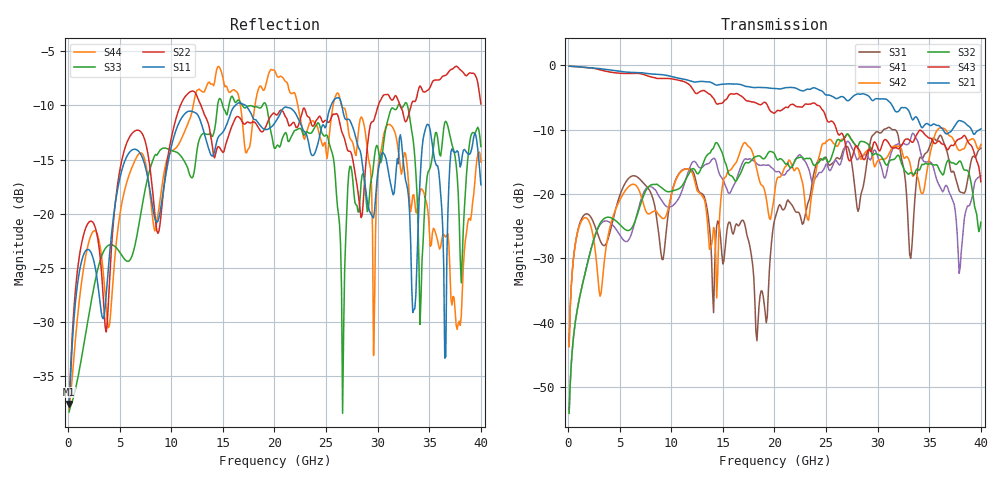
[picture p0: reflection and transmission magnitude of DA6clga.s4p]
! ADC12DJ3200QML-SP
! 196-pin ZMX package
! CLGA Ceramic Package without columns (ceramic land grid array)
! Texas Instruments 4/21/2021
! Single-ended  S-parameters
! PORT#  PORT_NAME  NET_NAME
! PORT1:  DAxN.DIEBUMP DAxN
! PORT2:  DAxN.BGA  DAxN
! PORT3:  DAxP.DIEBUMP DAxP
! PORT4:  DAxP.BGA  DAxP
! Touchstone Ver. 1.0
! Number of ports is 4
# Hz	S	MA	R	50.000000
! SCATTERING PARAMETERS  :
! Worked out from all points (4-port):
!   400 points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, 100 MHz to 40 GHz, reference 50 ohm
!   strongest paths, dB at 100 MHz, 10.1 GHz, 20.1 GHz, 30.1 GHz, 40 GHz:
!     S21: -0.1, -1.7, -3.6, -5.2, -9.9
!     S43: -0.1, -2.1, -7.3, -13.2, -18.1
!     S32: -54.1, -19.5, -14.1, -13.9, -24.4
!     S42: -43.7, -19.5, -18.7, -14.7, -12.3
!     S41: -54.1, -21.8, -16.5, -14.7, -17.1
!     S31: -43.7, -19.4, -23.5, -10.4, -12.9
!   lowest |S11| = -37.6 dB at 100 MHz (marker M1), VSWR 1.03, Z = 51.2 - j0.568 ohm
!   |S11| at or under -10 dB: start of sweep to 16.21 GHz; 17.21 GHz to 25.48 GHz (8.275 GHz wide, 38.8 % of centre); 26.52 GHz to end of sweep
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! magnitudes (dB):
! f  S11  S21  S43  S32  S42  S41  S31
! 100 MHz  -37.6  -0.1  -0.1  -54.1  -43.7  -54.1  -43.7
! 3 GHz  -27.4  -0.5  -0.6  -24.9  -34.9  -25.0  -26.8
! 14.3 GHz  -13.8  -3.0  -5.8  -12.0  -29.3  -14.7  -27.3
! 25.1 GHz  -11.3  -4.6  -8.5  -14.8  -11.7  -15.4  -14.7
! 26.6 GHz  -10.4  -4.9  -10.7  -11.6  -11.4  -14.1  -13.4
! 29.6 GHz  -20.4  -5.4  -12.0  -13.9  -15.2  -13.3  -10.8
! 40 GHz  -17.3  -9.9  -18.1  -24.4  -12.3  -17.1  -12.9
